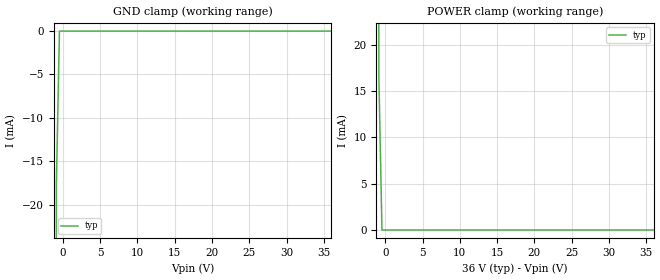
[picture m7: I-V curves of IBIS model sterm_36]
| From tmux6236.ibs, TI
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| sterm_36
[Model]   sterm_36
Model_type   Terminator
|   typ   min   max
C_comp   2.533030e-11   NA   NA
[Voltage Range]   36   NA   NA
[Temperature Range]   27   NA   NA
[Power Clamp Reference]   36   NA   NA
[GND Clamp Reference]   0   NA   NA
[GND Clamp]
|   Voltage   I(typ)   I(min)   I(max)
-5V       -7.155A    NA         NA
-1.273V   -346mA     NA         NA
-858.6mV  -17.64mA   NA         NA
-444.4mV  -1.252uA   NA         NA
36V       15.94nA    NA         NA
[POWER Clamp]
|   Voltage   I(typ)   I(min)   I(max)
-5V       7.404A     NA         NA
-1.273V   337.2mA    NA         NA
-858.6mV  16.5mA     NA         NA
-444.4mV  1.492uA    NA         NA
36V       -14.91nA   NA         NA
